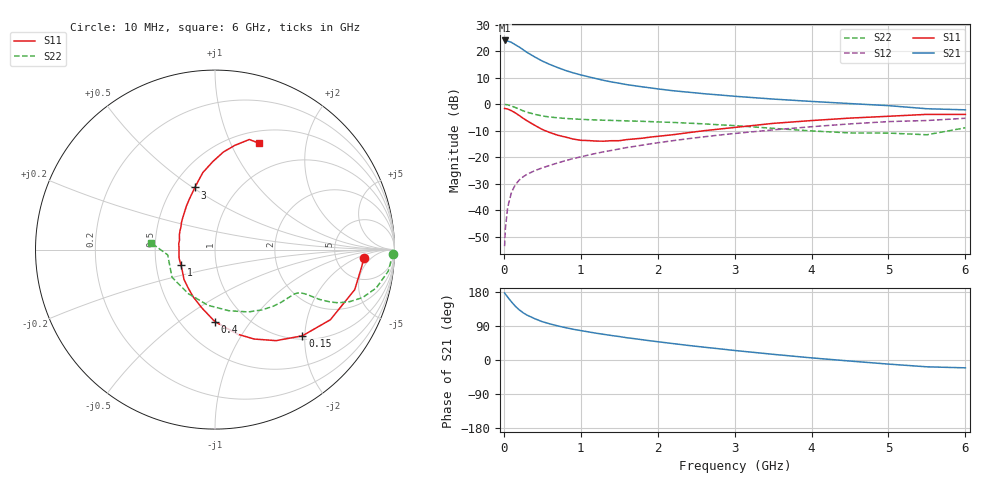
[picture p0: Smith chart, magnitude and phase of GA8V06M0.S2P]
! Infineon Technologies  Discrete & RF Semiconductors
! BF775
! Si NPN RF Bipolar Junction Transistor in SOT23
! VCE = 8 V  IC = 6 mA
! Common Emitter S-Parameters:  May  1996
# GHz  S  MA  R  50
!  f  S11  S21  S12  S22
! GHz  MAG  ANG  MAG  ANG  MAG  ANG  MAG  ANG
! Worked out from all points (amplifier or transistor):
!   36 points, 10 MHz to 6 GHz, reference 50 ohm
!   highest |S21| = 24.0 dB at 10 MHz (marker M1)
!   |S21| within 3 dB of that: start of sweep to 226.3 MHz
!   unconditionally stable (mu >= 1): 788.1 MHz to 2.994 GHz
!   at 250 MHz: K = 0.52, MSG = 24.0 dB, |S12| = -27.4 dB
!   at 1.4 GHz: K = 1.10, MAG = 10.9 dB, |S12| = -17.4 dB
!   at 6 GHz: K = 0.90, MSG = 1.6 dB, |S12| = -5.3 dB
!   S11 on the Smith chart (normalised r, x): 10 MHz: 10, -3; 150 MHz: 1.08, -1.95; 400 MHz: 0.72, -0.69; 1 GHz: 0.67, -0.12; 3 GHz: 0.64, +0.51; 6 GHz: 0.64, +1.29
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0.01  0.8301 -3.2  15.91 176.9  0.0021 83.5  0.9921 -1.3
0.02  0.8235 -6.4  15.57 173.8  0.0045 80.2  0.9851 -2.9
0.05  0.8099 -16.0  15.52 165.9  0.0114 80.5  0.973 -7.1
0.1  0.7522 -31.3  14.61 153.3  0.0219 73.2  0.9234 -13.4
0.15  0.684 -44.6  13.17 141.7  0.0304 68.3  0.8647 -18.0
0.2  0.6111 -56.1  11.96 132.4  0.0371 65.1  0.8051 -21.1
0.25  0.5437 -66.4  10.67 124.7  0.0426 61.8  0.7493 -23.3
0.3  0.488 -75.0  9.494 118.6  0.0474 61.2  0.7075 -24.4
0.4  0.4007 -90.2  7.805 109.2  0.0556 59.6  0.6446 -25.5
0.5  0.333 -102.7  6.503 101.1  0.063 59.4  0.5991 -25.8
0.6  0.2911 -114.4  5.594 95.2  0.0703 59.9  0.5718 -26.0
0.8  0.2401 -135.9  4.329 85.4  0.086 60.2  0.5382 -26.7
1  0.2084 -155.5  3.561 77.6  0.1016 61.3  0.5181 -27.9
1.1  0.2059 -166.4  3.283 74.2  0.1098 61.6  0.5101 -28.8
1.3  0.2005 178.7  2.808 67.7  0.1265 61.4  0.498 -30.8
1.6  0.215 157.6  2.333 58.7  0.1522 60.2  0.4838 -34.6
2.2  0.2657 130.3  1.793 43.3  0.2051 57.0  0.4525 -44.2
3  0.3638 108.0  1.41 25.1  0.2801 50.1  0.3943 -61.7
3.5  0.4343 99.0  1.248 15.0  0.3272 44.7  0.3501 -76.9
4.5  0.5464 85.0  1.026 -2.8  0.4248 32.6  0.2868 -121.3
5.5  0.6424 72.7  0.82 -18.0  0.4917 17.4  0.2649 -173.5
6  0.6416 67.4  0.782 -20.7  0.5423 13.2  0.3588 173.8
